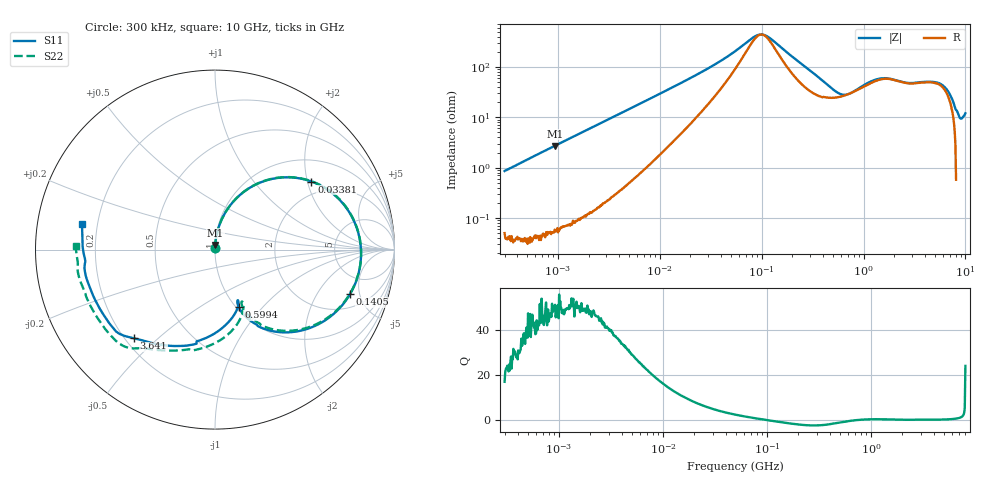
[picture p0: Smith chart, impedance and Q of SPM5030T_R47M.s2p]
! S-Parameter Data Generated by TDK Corporation
! Copyright(C) 2019 TDK Corporation.
! All Rights Reserved.
! TDK P/N: SPM5030T-R47M (Inductor)
! Property: L=470nH at 100kHz
! Size(LxWxT): 5.2x5x3mm
! Model Type: s2p (Touchstone File Format Version 1.0)
! Frequency: DC=Yes Start=0.3MHz Stop=10000MHz 802points Log-sweep
! Model Generated on Sep. 23, 2019
! Port Assignments:
!  1 ---@@@--- 2
! Applicable Conditions:
!  Temperature = 25 degC
!  DC Bias Current = 0 A
!  Small Signal Operation
! Terms and conditions regarding TDK Simulation Models
! (1)This simulation model is being provided solely for informational purposes. Please refer to the specifications of the products in terms of detailed characteristics of such products.
! (2)In no event shall TDK Corporation of any of its subsidiaries be liable for any loss or damage arising, directly or indirectly,
!  From any information contained in this simulation model, including, but not limited to loss or damages arising from any inaccuracies, omissions or errors in connection with such information.
! (3)Any and all copyrights on this simulation model are owned by TDK Corporation.
!  Duplication or redistribution of this simulation model without prior written permission from TDK Corporation is prohibited.
! (4)This simulation model is subject to any modification or change without any prior notice.
! (5)Neither TDK Corporation nor any of its subsidiaries shall make any warranty, express or implied,
!  Including but not limited to the correctness, implied warranties of merchantability and fitness for a particular purpose with respect to this simulation models.
! (6)The use of this simulation model shall be deemed to have consented to the terms and conditions hereof.
# Hz S MA R 50
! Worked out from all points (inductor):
!   801 points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, 300 kHz to 10 GHz, reference 50 ohm
!   read as one part in series: L = 457 nH near 318.3 kHz
!   highest Q = 50.9 at 930.3 kHz (marker M1), where L = 463 nH
!   self-resonance near 100.2 MHz
!   S11 on the Smith chart (normalised r, x): 300 kHz: 1.00, +0.02; 33.81 MHz: 1.58, +2.12; 140.5 MHz: 3.06, -4.06; 599.4 MHz: 1.03, -0.74; 3.641 GHz: 0.23, -0.42; 10 GHz: 0.14, +0.09
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300000  0.00817 85.4  0.9994 -0.5  0.9995 -0.5  0.008108 86.5
930288  0.02654 87.1  0.999 -1.6  0.9991 -1.6  0.02655 87.2
1713600  0.04897 85.9  0.9978 -2.9  0.9978 -2.9  0.04898 86.0
9671944  0.2642 70.8  0.9486 -15.7  0.9486 -15.7  0.2644 70.8
1.740512e7  0.4359 57.3  0.8541 -26.5  0.8541 -26.5  0.4363 57.3
3.38066e7  0.6575 35.2  0.6169 -41.4  0.6168 -41.4  0.6584 35.4
5.477226e7  0.7691 17.3  0.3821 -46.1  0.382 -46.1  0.77 17.5
9.561964e7  0.8145 -3.2  0.1865 -10.8  0.187 -10.6  0.8148 -2.9
1.405283e8  0.7927 -18.1  0.2706 28.3  0.2714 28.3  0.7927 -17.5
2.164412e8  0.7078 -36.3  0.4744 30.3  0.4749 30.2  0.7077 -35.4
3.126428e8  0.5837 -52.0  0.6348 18.8  0.635 18.7  0.5847 -50.6
4.448526e8  0.4415 -63.6  0.7265 3.5  0.7265 3.5  0.4459 -61.2
5.99416e8  0.3446 -67.6  0.7483 -10.9  0.7483 -10.9  0.3542 -64.4
1.024756e9  0.3352 -67.2  0.6476 -37.5  0.6477 -37.5  0.3621 -64.0
1.35547e9  0.402 -77.8  0.5448 -49.0  0.5449 -49.0  0.4466 -75.7
1.767019e9  0.4826 -93.3  0.4671 -56.7  0.4673 -56.7  0.5377 -93.7
2.720446e9  0.61 -119.6  0.3855 -75.8  0.3855 -75.9  0.6486 -120.6
3.640519e9  0.6701 -132.5  0.2975 -90.5  0.2977 -90.5  0.7041 -128.6
4.924213e9  0.7142 -140.1  0.2347 -102.0  0.2347 -102.0  0.7479 -136.0
6.172341e9  0.7187 -147.7  0.2053 -114.5  0.2054 -114.5  0.7555 -146.9
8.770142e9  0.7367 179.3  0.1418 -144.6  0.1418 -144.7  0.7738 -179.6
1e10  0.7527 169.1  0.1153 -151.2  0.115 -151.3  0.7754 178.3
